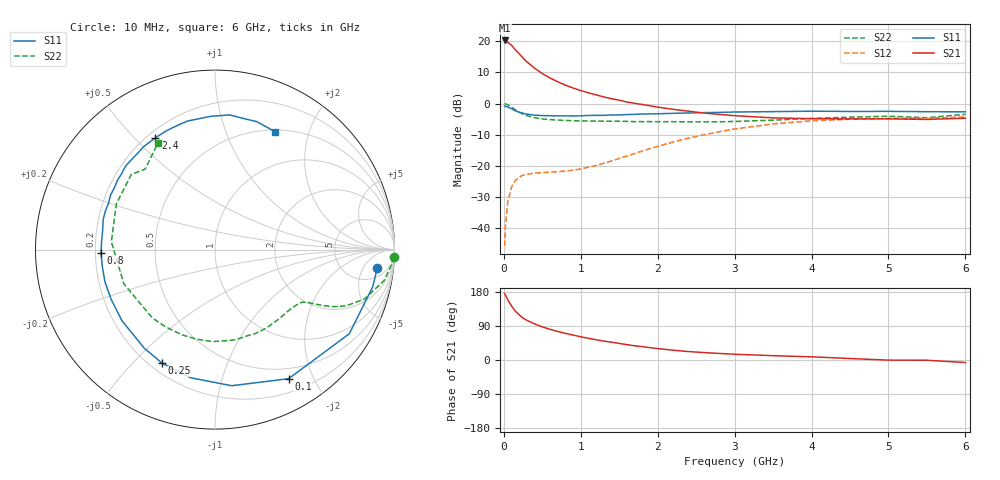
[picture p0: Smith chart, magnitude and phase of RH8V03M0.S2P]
! SIEMENS Small Signal Semiconductors
! BFR106
! Si NPN RF Bipolar Junction Transistor in SOT23
! VCE = 8 V  IC = 3 mA
! Common Emitter S-Parameters:  August  1996
# GHz  S  MA  R  50
!  f  S11  S21  S12  S22
! GHz  MAG  ANG  MAG  ANG  MAG  ANG  MAG  ANG
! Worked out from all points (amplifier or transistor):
!   36 points, 10 MHz to 6 GHz, reference 50 ohm
!   highest |S21| = 20.2 dB at 10 MHz (marker M1)
!   |S21| within 3 dB of that: start of sweep to 150.4 MHz
!   unconditionally stable (mu >= 1): 715.4 MHz to 1.794 GHz; 4.498 GHz to end of sweep
!   at 250 MHz: K = 0.38, MSG = 18.8 dB, |S12| = -22.9 dB
!   at 1.4 GHz: K = 1.18, MAG = 7.4 dB, |S12| = -18.4 dB
!   at 6 GHz: K = 1.02, MAG = -1.1 dB, |S12| = -4.3 dB
!   S11 on the Smith chart (normalised r, x): 10 MHz: 9, -10; 100 MHz: 0.36, -1.66; 250 MHz: 0.25, -0.61; 800 MHz: 0.22, -0.01; 2.4 GHz: 0.23, +0.58; 6 GHz: 0.52, +1.50
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0.01  0.9097 -6.5  10.25 175.1  0.0052 89.5  0.9975 -2.3
0.02  0.9032 -13.2  10.1 171.7  0.0107 82.3  0.9901 -4.4
0.05  0.8829 -32.1  9.643 159.1  0.0261 72.7  0.9578 -10.4
0.1  0.8279 -60.3  8.564 142.7  0.0461 60.0  0.8769 -18.3
0.15  0.7641 -83.0  7.264 128.6  0.0586 49.0  0.7941 -23.3
0.2  0.7269 -100.8  6.256 119.0  0.0663 43.1  0.7278 -25.9
0.25  0.6981 -114.9  5.358 110.6  0.0714 38.5  0.674 -27.5
0.3  0.6761 -125.7  4.645 104.7  0.0736 36.4  0.6402 -28.4
0.4  0.6525 -142.6  3.692 95.2  0.077 33.6  0.5937 -29.7
0.5  0.6417 -154.3  3.02 87.4  0.0781 33.6  0.5669 -31.1
0.6  0.639 -163.6  2.569 80.9  0.0798 35.2  0.5533 -33.2
0.8  0.6355 -178.3  1.973 70.4  0.083 41.5  0.5368 -38.0
1.1  0.6451 164.9  1.486 57.2  0.0955 54.1  0.5253 -47.1
1.6  0.6667 144.7  1.058 40.5  0.1445 68.1  0.5181 -65.0
2.2  0.6979 124.5  0.808 25.9  0.2421 68.2  0.5125 -91.0
2.4  0.7061 118.1  0.755 22.3  0.2796 65.7  0.5098 -101.3
3  0.7324 102.2  0.64 15.2  0.391 54.6  0.5167 -132.5
3.5  0.7427 92.0  0.59 11.4  0.4725 43.4  0.5423 -159.4
4.5  0.7472 77.3  0.569 3.9  0.561 21.2  0.6061 155.0
5  0.7502 72.0  0.569 -0.3  0.5781 12.4  0.6268 138.0
5.5  0.7406 66.7  0.557 -0.7  0.58 7.9  0.5935 131.0
6  0.7371 63.2  0.583 -6.7  0.6119 -0.3  0.6723 118.3
